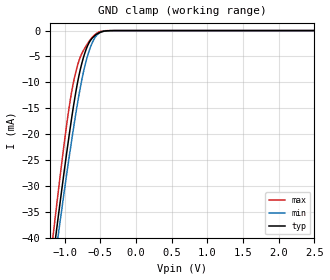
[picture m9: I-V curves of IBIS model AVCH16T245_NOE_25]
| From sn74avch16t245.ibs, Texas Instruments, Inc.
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[Model]   AVCH16T245_NOE_25
Model_type  Input
Vinl=0.7
Vinh=1.6
| variable   typ   min   max
C_comp   2.84pF   2.22pF   3.47pF
[Temperature Range]   40   100   -40
| Ambient temperature   25   85   -40
[Voltage range]   2.5   2.3   2.7
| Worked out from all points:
|   GND clamp passes 1 mA (typ) near -0.58 V on its own axis
[GND Clamp]
| AVCH16T245_NOE_25
|   Voltage   I(typ)   I(min)   I(max)
-4.6V     -463.5mA   -440.8mA   -490.1mA
-1.175V   -45.45mA   -48.4mA    -41.36mA
-1.145V   -42.15mA   -45.3mA    -37.79mA
-1.12V    -39.42mA   -42.73mA   -34.85mA
-1.095V   -36.71mA   -40.18mA   -31.93mA
-1.07V    -34.03mA   -37.66mA   -29.06mA
-945mV    -21.15mA   -25.38mA   -15.71mA
-840mV    -11.71mA   -15.87mA   -7.878mA
-760mV    -6.442mA   -9.645mA   -4.497mA
-685mV    -3.184mA   -5.238mA   -2.675mA
-520mV    -460.2uA   -539.6uA   -292.7uA
2.5V      198.5pA    973.5pA    43.42pA
